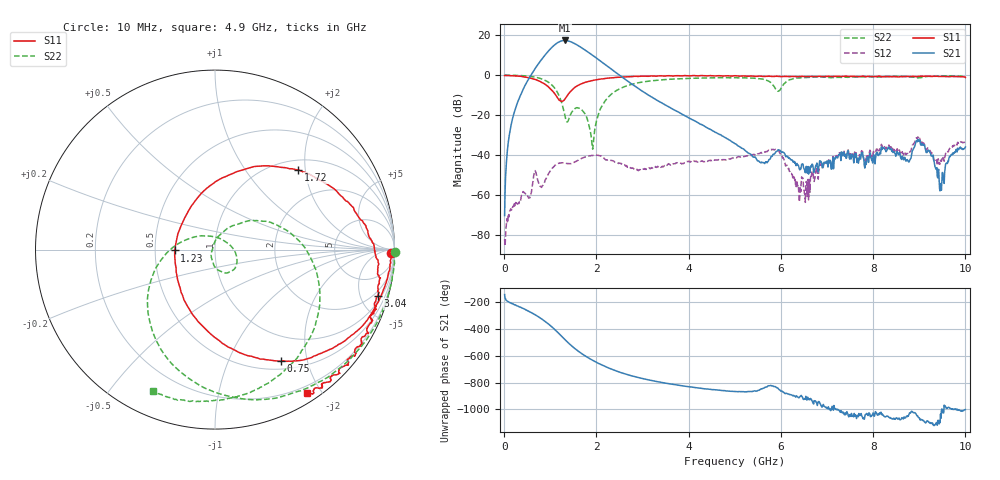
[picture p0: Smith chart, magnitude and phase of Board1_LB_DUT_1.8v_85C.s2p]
! Created Tue May 27 16:25:40 2025
# hz S ma R 50
! 2 Port Network Data from SP1.SP block
! freq  magS11  angS11  magS21  angS21  magS12  angS12  magS22  angS22
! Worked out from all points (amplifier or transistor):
!   1000 points, 10 MHz to 10 GHz, reference 50 ohm
!   highest |S21| = 17.4 dB at 1.31 GHz (marker M1)
!   |S21| within 3 dB of that: 1.056 GHz to 1.634 GHz (578.7 MHz wide, 43 % of centre)
!   unconditionally stable (mu >= 1): 19.91 MHz to 21.16 MHz; 57.91 MHz to 63.24 MHz; 115.7 MHz to end of sweep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
!   at 1.67 GHz: K = 7.87, MAG = 15.9 dB, |S12| = -41.9 dB
!   at 5.01 GHz: K = 45.09, MAG = -16.1 dB, |S12| = -41.2 dB
!   at 10 GHz: K = 54.06, MAG = -21.8 dB, |S12| = -33.1 dB
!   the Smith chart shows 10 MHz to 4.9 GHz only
!   S11 on the Smith chart (normalised r, x): 10 MHz: 53, -45; 750 MHz: 0.61, -1.58; 1.23 GHz: 0.63, -0.01; 1.72 GHz: 1.21, +1.84; 3.04 GHz: 1.42, -6.89; 4.9 GHz: 0.11, -1.83
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1e7  0.9782 -1.1  0.0003025 -143.0  7.677e-05 136.0  1.005 -0.8
2e8  0.9638 -13.7  0.09796 145.9  0.0005309 71.8  0.9958 -17.8
7.5e8  0.7223 -59.6  1.977 49.3  0.001952 61.6  0.8512 -78.4
9.1e8  0.5665 -79.5  3.449 11.2  0.002552 109.3  0.7195 -103.6
1.05e9  0.3996 -105.3  5.182 -28.7  0.004764 98.6  0.5444 -131.7
1.14e9  0.2898 -131.9  6.316 -57.5  0.005898 84.8  0.3967 -154.3
1.23e9  0.224 -178.8  7.147 -88.4  0.006336 70.9  0.234 176.8
1.31e9  0.2447 133.4  7.423 -116.2  0.006277 62.4  0.1075 134.3
1.47e9  0.4233 79.3  6.69 -167.8  0.006152 58.9  0.1198 -12.9
1.68e9  0.6131 47.3  4.851 136.9  0.008225 51.1  0.1371 -68.9
1.72e9  0.6433 43.7  4.526 127.8  0.00854 47.8  0.12 -78.1
1.91e9  0.7368 28.2  3.195 88.4  0.009696 29.0  0.01595 -168.0
2.11e9  0.8063 16.7  2.168 53.0  0.009387 5.7  0.1614 54.5
2.48e9  0.8872 0.6  1.042 1.0  0.00611 -7.3  0.4411 10.7
3.04e9  0.9451 -15.9  0.3685 -52.4  0.00453 6.1  0.685 -33.7
3.34e9  0.9536 -24.1  0.2259 -73.7  0.004997 9.5  0.7516 -51.4
4.9e9  0.9518 -57.2  0.02321 -144.1  0.007913 -7.0  0.8619 -113.7
5.01e9  0.9697 -59.4  0.01915 -145.7  0.008703 -10.4  0.8622 -117.6
6.67e9  0.9336 -90.4  0.005805 148.8  0.003654 145.2  0.8906 -149.8
8.34e9  0.9165 -134.9  0.01588 22.3  0.0177 32.2  0.9216 172.9
9.49e9  0.9316 -167.2  0.002156 84.3  0.00763 67.2  0.953 164.5
1e10  0.8747 178.3  0.0158 79.5  0.02225 72.1  0.9168 163.8
